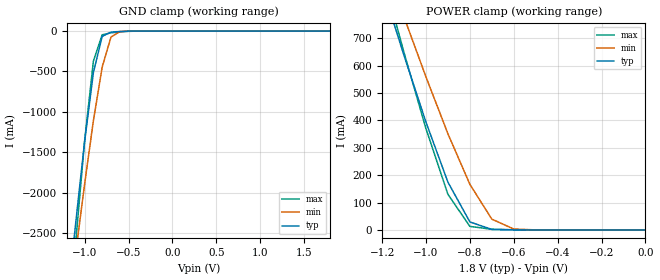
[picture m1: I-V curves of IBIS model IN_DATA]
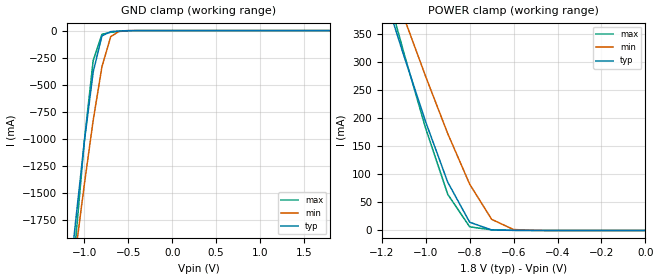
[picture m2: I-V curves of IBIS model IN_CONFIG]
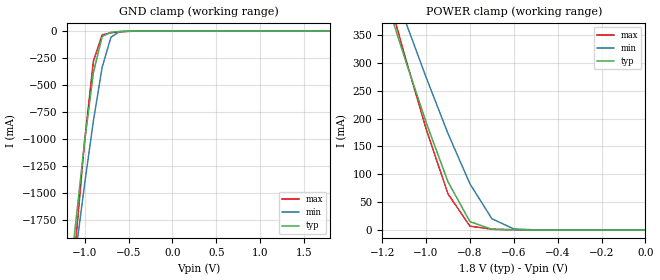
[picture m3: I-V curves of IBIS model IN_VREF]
| IBIS file 4pw864dy_c_t.ibs created by s2ibis2 version 1.2
| North Carolina State University Electronics Research Laboratory  1995
[IBIS ver]   2.1
[File name]   4pw864dy_c_t.ibs
[File Rev]   1.0
[Date]   Friday, March 12, 2004
[Source]   IDT
[Notes]   1. Temp typ=25C, min=0C, max=110C
   2. IDT C11.5 1.8V 1P 2-6M process
   3. Ramp rates based on 10Gig ohm load
   *** Important Notes ***
This IBIS file is for the 1:1 Registered Buffer with configuration settings
C0=0, C1=0 (Type C)
[Disclaimer]
READ THESE TERMS AND CONDITIONS CAREFULLY BEFORE USING THIS IBIS MODEL.  BY
USING THIS IBIS MODEL, YOU ARE ACCEPTING AND AGREEING TO THESE TERMS AND
CONDITIONS OF USE.
Integrated Device Technology, Inc. ("IDT") hereby grants the user of this
IBIS model ("User") a non-exclusive, nontransferable license to use this
IBIS model under the following terms: The User is granted this license only
to use the IBIS model for demonstration purposes only and is not granted
rights to sell, copy (except as needed to run the IBIS model), rent, lease
or sub-license (except for demonstration) the IBIS model in whole or in
part, or in modified form to anyone. The User may modify the IBIS model to
suit its specific applications, but  rights to derivative works and such
modifications shall belong to IDT.
THIS IBIS MODEL IS PROVIDED ON AN AS IS" BASIS AND IDT  MAKES ABSOLUTELY NO
WARRANTY WITH RESPECT TO THE INFORMATION CONTAINED HEREIN.  IDT DISCLAIMS
AND USER WAIVES ALL WARRANTIES, EXPRESS AND IMPLIED, INCLUDING WARRANTIES OF
MERCHANTABILITY AND FITNESS FOR A PARTICULAR PURPOSE.  THE ENTIRE RISK AS TO
QUALITY AND PERFORMANCE IS WITH THE USER  ACCORDINGLY, IN NO EVENT SHALL IDT
BE LIABLE FOR ANY DIRECT OR INDIRECT DAMAGES, WHETHER IN CONTRACT OR TORT,
INCLUDING ANY LOST PROFITS OR OTHER INCIDENTAL, CONSEQUENTIAL, EXEMPLARY, OR
PUNITIVE DAMAGES ARISING OUT OF THE USE OR APPLICATION OF THE  IBIS MODEL,
WHETHER OR NOT IDT HAD NOTICE OF SUCH DAMAGES.
IDT reserves the right to make changes without notice to any product herein
to improve reliability, function, or design. IDT does not convey any license
under patent rights or any other intellectual property rights, including
those of third parties. IDT is not obligated to provide  maintenance or
support for the licensed IBIS model.
This model is IDT74SSTU32864C 1:1 Registered Buffer with 1.8 SSTL I/O
[Copyright]
Copyright 2002, Integrated Device Technology, Inc. All rights
reserved.
|   Component IDT4PW864DY
[Component]   IDT4PW864DY
[Manufacturer]   Integrated Device Technology, Inc.
[Package]
| variable   typ   min   max
R_pkg   0.01480   0.01480   0.01480
L_pkg   1.05000nH   1.05000nH   1.05000nH
C_pkg   0.29100pF   0.29100pF   0.29100pF
[Pin]  signal_name   model_name   R_pin   L_pin   C_pin
A1   DCKE   IN_DATA
A2   NC   NC
A3   VREF   IN_VREF
A4   VDD   POWER
A5   QCKE   OUTBUF
A6   NC   NC
B1   D2   IN_DATA
B2   D15   IN_DATA
B3   GND   GND
B4   GND   GND
B5   Q2   OUTBUF
B6   Q15   OUTBUF
C1   D3   IN_DATA
C2   D16   IN_DATA
C3   VDD   POWER
C4   VDD   POWER
C5   Q3   OUTBUF
C6   Q16   OUTBUF
D1   DODT   IN_DATA
D2   NC   NC
D3   GND   GND
D4   GND   GND
D5   QODT   OUTBUF
D6   NC   NC
E1   D5   IN_DATA
E2   D17   IN_DATA
E3   VDD   POWER
E4   VDD   POWER
E5   Q5   OUTBUF
E6   Q17   OUTBUF
F1   D6   IN_DATA
F2   D18   IN_DATA
F3   GND   GND
F4   GND   GND
F5   Q6   OUTBUF
F6   Q18   OUTBUF
G1   NC   NC
G2   _RESET_   IN_RESET
G3   VDD   POWER
G4   VDD   POWER
G5   C1   IN_CONFIG
G6   C0   IN_CONFIG
H1   CLK   IN_CLK
H2   _DCS_   IN_CSGATEN
H3   GND   GND
H4   GND   GND
H5   _QCS_   OUTBUF
H6   NC   NC
J1   _CLK_   IN_CLK
J2   _CSR_   IN_CSGATEN
J3   VDD   POWER
J4   VDD   POWER
J5   NC   NC
J6   NC   NC
K1   D8   IN_DATA
K2   D19   IN_DATA
K3   GND   GND
K4   GND   GND
K5   Q8   OUTBUF
K6   Q19   OUTBUF
L1   D9   IN_DATA
L2   D20   IN_DATA
L3   VDD   POWER
L4   VDD   POWER
L5   Q9   OUTBUF
L6   Q20   OUTBUF
M1   D10   IN_DATA
M2   D21   IN_DATA
M3   GND   GND
M4   GND   GND
M5   Q10   OUTBUF
M6   Q21   OUTBUF
N1   D11   IN_DATA
N2   D22   IN_DATA
N3   VDD   POWER
N4   VDD   POWER
N5   Q11   OUTBUF
N6   Q22   OUTBUF
P1   D12   IN_DATA
P2   D23   IN_DATA
P3   GND   GND
P4   GND   GND
P5   Q12   OUTBUF
P6   Q23   OUTBUF
R1   D13   IN_DATA
R2   D24   IN_DATA
R3   VDD   POWER
R4   VDD   POWER
R5   Q13   OUTBUF
R6   Q24   OUTBUF
T1   D14   IN_DATA
T2   D25   IN_DATA
T3   VREF   IN_VREF
T4   VDD   POWER
T5   Q14   OUTBUF
T6   Q25   OUTBUF
| d   d   dummy_model
| din  din   dummy_model
[Diff Pin]  inv_pin   vdiff   tdelay_typ  tdelay_min  tdelay_max
H1   J1   0.60000V  NA   |CLK<P:N> Input  Pair
| Models and submodels in the file (7): IN_DATA (Input), IN_CONFIG (Input), IN_VREF (Input), IN_CLK (Input), IN_CSGATEN (Input), IN_RESET (Input), OUTBUF (Output)
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|   Model IN_DATA
[Model]   IN_DATA
Model_type   Input
Vinl =  0.65000V
Vinh =  1.15000V
C_comp   2.50000pF   2.50000pF   2.50000pF
[Temperature Range]   25.00000   0.11000k   0.000
[Voltage Range]   1.80000V   1.70000V   1.90000V
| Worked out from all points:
|   GND clamp passes 1 mA (typ) near -0.50 V on its own axis
|   POWER clamp passes 1 mA (typ) near -0.64 V on its own axis
[GND_clamp]
| voltage   I(typ)   I(min)   I(max)
-1.8V     -10.01A    -9.034A    -12.29A
-1.2V     -3.402A    -3.598A    -3.91A
-1.1V     -2.357A    -2.731A    -2.591A
-1V       -1.366A    -1.893A    -1.357A
-900mV    -512.4mA   -1.108A    -371.9mA
-800mV    -65.6mA    -445.2mA   -46.17mA
-700mV    -12.81mA   -74.32mA   -21.4mA
-600mV    -4.632mA   -6.378mA   -10.47mA
-400mV    -151.1uA   -107.5uA   -515.4uA
1.8V      13.82nA    12.76nA    492.7pA
[POWER_clamp]
| voltage   I(typ)   I(min)   I(max)
-1.8V     2.486A     2.403A     2.783A
-1.2V     891mA      1.002A     940.1mA
-1.1V     637mA      777.5mA    647.6mA
-1V       393.6mA    558.9mA    369.7mA
-900mV    174.5mA    351.3mA    130.1mA
-800mV    29.33mA    166.7mA    13.12mA
-700mV    1.951mA    39.57mA    2.484mA
-600mV    305.6uA    3.357mA    798.8uA
-500mV    48.35uA    239.3uA    163.9uA
0V        857.4pA    662pA      637.7pA
|   Model IN_CONFIG
[Model]   IN_CONFIG
Model_type   Input
Vinl =  0.000V
Vinh =  1.80000V
C_comp   1.750000pF   1.75000pF   1.75000pF
[Temperature Range]   25.00000   0.11000k   0.000
[Voltage Range]   1.80000V   1.70000V   1.90000V
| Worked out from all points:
|   GND clamp passes 1 mA (typ) near -0.51 V on its own axis
|   POWER clamp passes 1 mA (typ) near -0.70 V on its own axis
[GND_clamp]
| voltage   I(typ)   I(min)   I(max)
-1.8V     -7.509A    -6.777A    -9.219A
-1.2V     -2.552A    -2.699A    -2.933A
-1.1V     -1.768A    -2.049A    -1.943A
-1V       -1.025A    -1.42A     -1.018A
-900mV    -384.3mA   -831.8mA   -278.9mA
-800mV    -49.16mA   -334.1mA   -34.6mA
-700mV    -9.52mA    -55.82mA   -15.97mA
-600mV    -3.358mA   -4.767mA   -7.725mA
-400mV    -53.67uA   -34.09uA   -242.5uA
1.8V      26.95pA    5.248nA    -19.88pA
[POWER_clamp]
| voltage   I(typ)   I(min)   I(max)
-1.8V     1.209A     1.169A     1.353A
-1.2V     434.4mA    488.7mA    458.3mA
-1.1V     311.1mA    379.5mA    316.3mA
-1V       192.7mA    273.3mA    181mA
-900mV    85.9mA     172.3mA    64.37mA
-800mV    14.67mA    82.28mA    6.452mA
-700mV    926.3uA    19.77mA    1.156mA
-600mV    137.1uA    1.636mA    359.6uA
-500mV    21.08uA    107.7uA    70.28uA
0V        26.95pA    124.4pA    8.257pA
|   Model IN_VREF
[Model]   IN_VREF
Model_type   Input
Vinl =  0.83300V
Vinh =  0.96900V
C_comp   1.750000pF   1.75000pF   1.75000pF
[Temperature Range]   25.00000   0.11000k   0.000
[Voltage Range]   1.80000V   1.70000V   1.90000V
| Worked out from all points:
|   GND clamp passes 1 mA (typ) near -0.50 V on its own axis
|   POWER clamp passes 1 mA (typ) near -0.69 V on its own axis
[GND_clamp]
| voltage   I(typ)   I(min)   I(max)
-1.8V     -7.51A     -6.777A    -9.22A
-1.2V     -2.552A    -2.7A      -2.934A
-1.1V     -1.768A    -2.049A    -1.944A
-1V       -1.025A    -1.42A     -1.018A
-900mV    -385mA     -832.1mA   -279.5mA
-800mV    -49.71mA   -334.4mA   -35.16mA
-700mV    -10.01mA   -56.13mA   -16.48mA
-600mV    -3.774mA   -5.075mA   -8.176mA
-300mV    -47.02uA   -56.45uA   -126.6uA
1.8V      49.15nA    26.41nA    5.103nA
[POWER_clamp]
| voltage   I(typ)   I(min)   I(max)
-1.8V     1.213A     1.173A     1.357A
-1.2V     436.1mA    490.7mA    459.9mA
-1.1V     312.4mA    381.2mA    317.5mA
-1V       193.7mA    274.6mA    182mA
-900mV    86.67mA    173.3mA    64.98mA
-800mV    15.07mA    83.05mA    6.858mA
-700mV    1.114mA    20.26mA    1.39mA
-600mV    207.8uA    1.878mA    482.9uA
-500mV    38.54uA    180.7uA    114.2uA
0V        5.276nA    15.76nA    22.22nA
